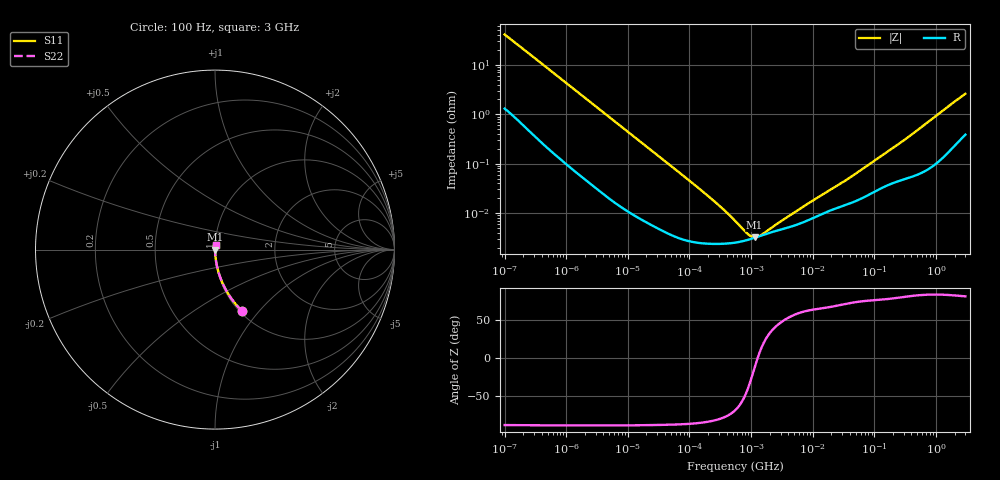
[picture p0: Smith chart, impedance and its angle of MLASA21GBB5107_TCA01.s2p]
! MLASA21GBB5107_TCA01  S-PARAMETER MODEL  ( Standard Model )
! Model Generated by TAIYO YUDEN Corporation (http://www.ty-top.com)
! Version 1.0
! TAIYO YUDEN Control No. 220601
! Copyright(c) 2019 TAIYO YUDEN CO.,LTD. All Rights Reserved.
! Product Description (link to TY-COMPAS)
! https://ds.yuden.co.jp/TYCOMPAS/or/detail?pn=MLASA21GBB5107MTCA01&u=M
! Products Name : Multilayer Ceramic Capacitors
! Characteristics :
!  Capacitance : 100 [uF] , Rated Voltage : 4 [V] , TCC : X5R
!  Case Size : 2.0 x 1.25 / 0.079 x 0.049 [mm/inch] , Thickness : 1.25 / 0.049 [mm/inch]
!  (Conditions: Temperature = 25 [degC] , DC Bias Voltage = 0 [V])
! External Node Assignments :
!  1  o---| |---o  2
! GND o---------o GND
! Frequency Range : 100Hz  -  3GHz  [ 401 STEP ]
# MHZ S RI R 50
! Freq[MHz].  S11 Real  S11 Imag  S21 Real  S21 Imag  S12 Real  S12 Imag  S22 Real  S22 Imag
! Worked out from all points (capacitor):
!   401 points, 100 Hz to 3 GHz, reference 50 ohm
!   read as one part in series: C = 38.4 uF near 109 Hz
!   lowest |Z| = 3.24 mohm at 1.139 MHz (marker M1)
!   series resonance near 1.275 MHz, so ESL is about 410 pH
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0.0001  0.1528 -0.3443  0.8472 0.3443  0.8472 0.3443  0.1528 -0.3443
0.000114  0.1241 -0.3144  0.8759 0.3144  0.8759 0.3144  0.1241 -0.3144
0.000175  0.0597 -0.2226  0.9403 0.2226  0.9403 0.2226  0.0597 -0.2226
0.000348  0.0174 -0.1187  0.9826 0.1187  0.9826 0.1187  0.0174 -0.1187
0.000724  0.00481 -0.0586  0.9952 0.0586  0.9952 0.0586  0.00481 -0.0586
0.001788  0.00112 -0.0241  0.9989 0.0241  0.9989 0.0241  0.00112 -0.0241
0.005476  0.000243 -0.008  0.9998 0.008  0.9998 0.008  0.000243 -0.008
0.031977  4.94e-05 -0.0014  1 0.0014  1 0.0014  4.94e-05 -0.0014
0.157206  2.46e-05 -0.000284  1 0.000284  1 0.000284  2.46e-05 -0.000284
0.388167  2.41e-05 -0.000104  1 0.000104  1 0.000104  2.41e-05 -0.000104
0.441669  2.44e-05 -8.85e-05  1 8.85e-05  1 8.85e-05  2.44e-05 -8.85e-05
0.547723  2.52e-05 -6.53e-05  1 6.53e-05  1 6.53e-05  2.52e-05 -6.53e-05
1.138514  3.16e-05 -7.07e-06  1 7.07e-06  1 7.07e-06  3.16e-05 -7.07e-06
4.711951  5.43e-05 8.09e-05  0.9999 -8.09e-05  0.9999 -8.09e-05  5.43e-05 8.09e-05
5.361412  5.73e-05 9.19e-05  0.9999 -9.19e-05  0.9999 -9.19e-05  5.73e-05 9.19e-05
9.794414  7.79e-05 0.000158  0.9999 -0.000158  0.9999 -0.000158  7.79e-05 0.000158
34.12477  0.000146 0.000434  0.9999 -0.000434  0.9999 -0.000434  0.000146 0.000434
175.1444  0.00038 0.0018  0.9996 -0.0018  0.9996 -0.0018  0.00038 0.0018
396.7889  0.00055 0.00379  0.9994 -0.00379  0.9994 -0.00379  0.00055 0.00379
2036.508  0.00266 0.018  0.9973 -0.018  0.9973 -0.018  0.00266 0.018
2752.553  0.00402 0.0236  0.996 -0.0236  0.996 -0.0236  0.00402 0.0236
3000  0.0045 0.0255  0.9955 -0.0255  0.9955 -0.0255  0.0045 0.0255
